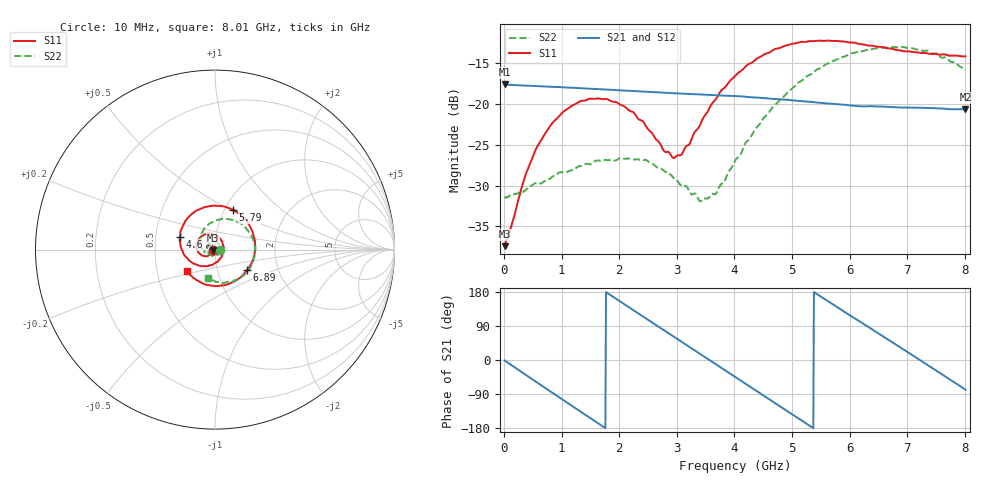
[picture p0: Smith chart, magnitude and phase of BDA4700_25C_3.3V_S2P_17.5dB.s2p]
!Agilent Technologies,E5071B,MY42404982,A.09.10
!Date: Mon Oct 20 18:10:23 2025
!Data & Calibration Information:
!Freq	S11:SOLT2(ON)	S21:SOLT2(ON)	S12:SOLT2(ON)	S22:SOLT2(ON)
# Hz S RI R 50
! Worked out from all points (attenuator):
!   801 points, 10 MHz to 8.01 GHz, reference 50 ohm
!   highest |S21| = -17.59 dB at 10 MHz (marker M1); lowest = -20.7 dB at 8.01 GHz (marker M2)
!   lowest |S11| = -37.4 dB at 10 MHz (marker M3), VSWR 1.03, Z = 48.7 - j0.141 ohm
!   |S11| at or under -10 dB: start of sweep to end of sweep
!   |S22| runs from -31.9 to -13.0 dB; largest |S21 - S12| = 0.0015
!   S11 on the Smith chart (normalised r, x): 10 MHz: 0.97, -0.00; 4.6 GHz: 0.67, +0.10; 5.79 GHz: 1.10, +0.52; 6.89 GHz: 1.39, -0.33; 8.01 GHz: 0.71, -0.18
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1e7  -0.0134 -0.00145  0.1319 -0.00287  0.1319 -0.00295  0.0268 -0.000846
3.6e8  -0.0242 -0.0261  0.1031 -0.079  0.1031 -0.079  0.0225 -0.019
5.8e8  -0.0416 -0.0362  0.0644 -0.1116  0.0645 -0.1116  0.0142 -0.0293
8.7e8  -0.0712 -0.0333  0.000938 -0.1275  0.000927 -0.1275  -0.00696 -0.0357
1.35e9  -0.1038 0.0137  -0.0934 -0.0831  -0.0934 -0.0832  -0.038 -0.0173
1.77e9  -0.0826 0.0687  -0.1228 0.00166  -0.1228 0.00169  -0.0428 0.0151
2.07e9  -0.042 0.0881  -0.1039 0.0623  -0.1039 0.0623  -0.0291 0.0361
2.68e9  0.04 0.0432  0.00382 0.1179  0.00363 0.1178  0.0169 0.037
2.93e9  0.0469 0.000526  0.0524 0.1043  0.0523 0.104  0.0278 0.0222
3.05e9  0.0437 -0.021  0.0727 0.0906  0.0719 0.091  0.0296 0.0125
3.42e9  -0.00262 -0.0769  0.1109 0.029  0.111 0.029  0.0195 -0.0163
3.68e9  -0.0555 -0.092  0.1111 -0.022  0.1112 -0.0223  2.74e-05 -0.0282
4.01e9  -0.1308 -0.0702  0.0803 -0.0781  0.0804 -0.0779  -0.0352 -0.0273
4.6e9  -0.1942 0.0706  -0.0249 -0.1053  -0.0247 -0.1054  -0.081 0.0368
4.95e9  -0.157 0.1702  -0.0789 -0.0706  -0.0787 -0.0712  -0.0715 0.0962
5.35e9  -0.0472 0.2387  -0.1029 -0.00382  -0.1028 -0.00443  -0.0141 0.1529
5.79e9  0.1015 0.2217  -0.0753 0.0655  -0.0751 0.0655  0.0872 0.1671
6.24e9  0.2064 0.1064  -0.00978 0.0963  -0.00825 0.0965  0.1847 0.1037
6.68e9  0.214 -0.0479  0.0585 0.0762  0.0587 0.0762  0.222 -0.00863
6.89e9  0.1799 -0.114  0.0805 0.0507  0.0808 0.0503  0.2124 -0.0683
7.45e9  0.00844 -0.2036  0.087 -0.0366  0.087 -0.0368  0.1041 -0.1741
8.01e9  -0.1553 -0.1203  0.0189 -0.0908  0.0193 -0.0909  -0.0374 -0.1569
